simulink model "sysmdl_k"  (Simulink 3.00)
settings: Solver=ode45  SolverMode=SingleTasking  StartTime=0.0  StopTime=10.0  RelTol=1e-3  AbsTol=1e-6
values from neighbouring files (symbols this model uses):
  g = 9.8    [ch8_c.m]    (also in ch8_d.m; ch8_h.m; s_xmp2.m)
  I_m = 0.75    [ch8_h.m]
  l = sqrt(dx1^2 + dx2^2)*7.5    [ch8_b.m]    (also in ch8_c.m = 0.5; ch8_d.m = 0.5; ch8_f.m; ch8_h.m = 0.3)
  m = 0.1    [ch8_c.m]    (also in ch8_d.m; ch8_h.m = 0.2; s_xmp3.m = 1; auto_param.m = 500)

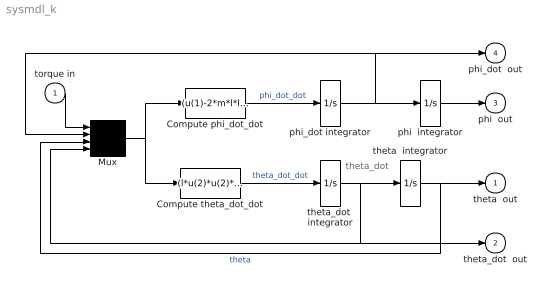
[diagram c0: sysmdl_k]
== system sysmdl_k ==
  note: theta_dot
  torque in : Inport  Port=1  PortWidth=-1  SampleTime=-1  DataType=auto
  Compute phi_dot_dot : Fcn  Expr=(u(1)-2*m*l*l*u(2)*u(4)*sin(u(3))*cos(u(3)))/(I_m+m*l*l*sin(u(3))*sin(u(3)))
  Compute theta_dot_dot : Fcn  Expr=(l*u(2)*u(2)*cos(u(3))-g)*sin(u(3))/l
  Mux : Mux  Inputs=4
  phi  integrator : Integrator  ExternalReset=none  InitialConditionSource=internal  InitialCondition=0  LimitOutput=off  UpperSaturationLimit=inf  LowerSaturationLimit=-inf  ShowSaturationPort=off  ShowStatePort=off  AbsoluteTolerance=auto
  phi_dot integrator : Integrator  ExternalReset=none  InitialConditionSource=internal  InitialCondition=0  LimitOutput=off  UpperSaturationLimit=inf  LowerSaturationLimit=-inf  ShowSaturationPort=off  ShowStatePort=off  AbsoluteTolerance=auto
  theta  integrator : Integrator  ExternalReset=none  InitialConditionSource=internal  InitialCondition=0  LimitOutput=off  UpperSaturationLimit=inf  LowerSaturationLimit=-inf  ShowSaturationPort=off  ShowStatePort=off  AbsoluteTolerance=auto
  theta_dot  integrator : Integrator  ExternalReset=none  InitialConditionSource=internal  InitialCondition=0  LimitOutput=off  UpperSaturationLimit=inf  LowerSaturationLimit=-inf  ShowSaturationPort=off  ShowStatePort=off  AbsoluteTolerance=auto
  theta  out : Outport  Port=1  InitialOutput=0
  theta_dot  out : Outport  Port=2  InitialOutput=0
  phi  out : Outport  Port=3  InitialOutput=0
  phi_dot  out : Outport  Port=4  InitialOutput=0
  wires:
  phi_dot integrator/1 -> phi  integrator/1, Mux/2, phi_dot  out/1
  theta_dot  integrator/1 -> theta  integrator/1, Mux/4, theta_dot  out/1
  theta  integrator/1 -> theta  out/1, Mux/3  "theta"
  torque in/1 -> Mux/1
  Compute phi_dot_dot/1 -> phi_dot integrator/1  "phi_dot_dot"
  Compute theta_dot_dot/1 -> theta_dot  integrator/1  "theta_dot_dot"
  Mux/1 -> Compute theta_dot_dot/1, Compute phi_dot_dot/1
  phi  integrator/1 -> phi  out/1
